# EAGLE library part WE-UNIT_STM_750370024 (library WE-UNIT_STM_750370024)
Off-Line Transformer WE-Unit STM - Nominal input voltage: 85-265 VAC - Operating temperature: -40°C to +125 °C - Isolation voltage 4 kVAC -- Especially designed for several ICs from STMicroelectronics VIPer 17H -- Universal input -- Offline-switch mode power supplies
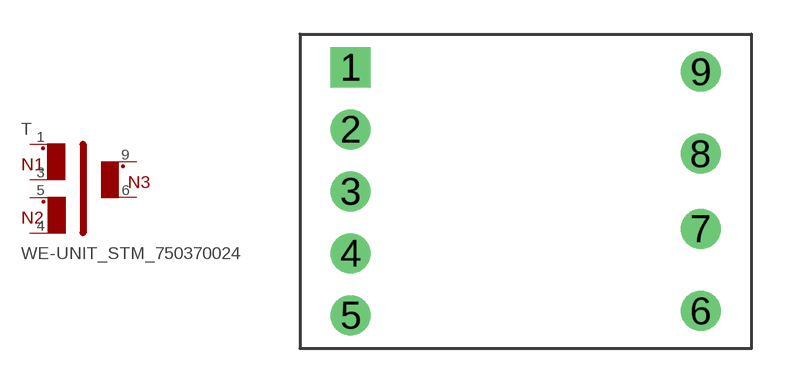
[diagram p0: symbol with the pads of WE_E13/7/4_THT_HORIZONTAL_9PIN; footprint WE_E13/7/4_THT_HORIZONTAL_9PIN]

Designator prefix T

## WE-UNIT_STM_750370024 (MPN: 750370024; OC_FARNELL: 1849042; OC_NEWARK: 13T9835; PACKAGE: EE13/7/4; SUPPLIER: Würth Elektronik eiSos GmbH)  [WE_E13/7/4_THT_HORIZONTAL_9PIN]
1  1  pas
3  2  pas
4  4  pas
5  3  pas
6  5  pas
9  6  pas

## Footprint WE_E13/7/4_THT_HORIZONTAL_9PIN (pad centres in mm)
Transformer, E13/7/4 THT Horizontal 9 Pin
drill 1.17 square: 1 -7.675,5.44
drill 1.17: 2 -7.675,2.72; 3 -7.675,0; 4 -7.675,-2.72; 5 -7.675,-5.44; 6 7.675,-5.25; 7 7.675,-1.65; 8 7.675,1.65; 9 7.675,5.25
